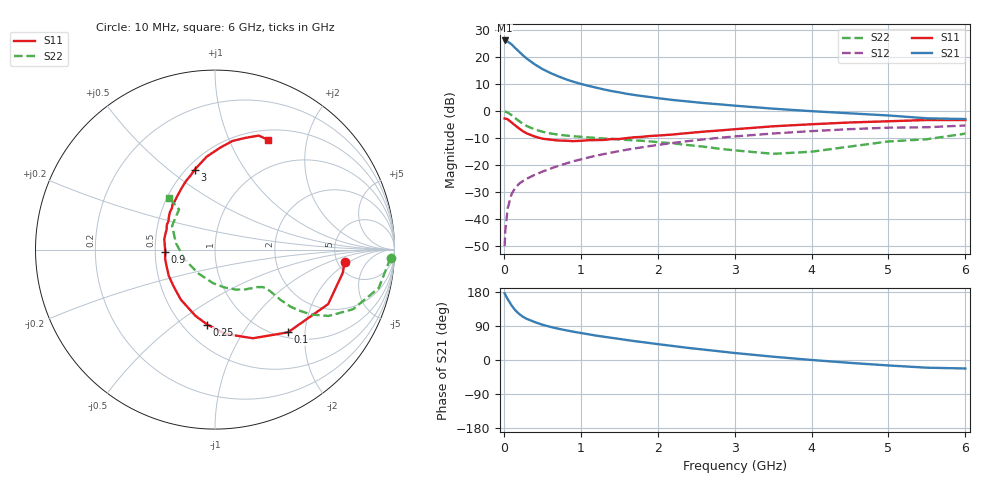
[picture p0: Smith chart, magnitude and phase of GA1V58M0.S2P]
! Infineon Technologies  Discrete & RF Semiconductors
! BF775
! Si NPN RF Bipolar Junction Transistor in SOT23
! VCE = 1.5 V  IC = 8 mA
! Common Emitter S-Parameters:  May  1996
# GHz  S  MA  R  50
!  f  S11  S21  S12  S22
! GHz  MAG  ANG  MAG  ANG  MAG  ANG  MAG  ANG
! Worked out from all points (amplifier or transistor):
!   36 points, 10 MHz to 6 GHz, reference 50 ohm
!   highest |S21| = 26.0 dB at 10 MHz (marker M1)
!   |S21| within 3 dB of that: start of sweep to 155.9 MHz
!   unconditionally stable (mu >= 1): 580.8 MHz to 4.246 GHz; 5.163 GHz to end of sweep
!   at 250 MHz: K = 0.65, MSG = 23.1 dB, |S12| = -25.8 dB
!   at 1.4 GHz: K = 1.14, MAG = 9.0 dB, |S12| = -15.4 dB
!   at 6 GHz: K = 1.00, MAG = 0.9 dB, |S12| = -5.4 dB
!   S11 on the Smith chart (normalised r, x): 10 MHz: 5.82, -1.65; 100 MHz: 1.10, -1.63; 250 MHz: 0.65, -0.66; 900 MHz: 0.57, -0.02; 3 GHz: 0.55, +0.62; 6 GHz: 0.62, +1.41
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0.01  0.7259 -5.3  19.96 176.0  0.0032 91.1  0.9804 -2.7
0.02  0.7233 -10.4  19.72 171.8  0.0064 85.4  0.9646 -5.4
0.05  0.6999 -25.7  19.03 160.6  0.016 77.7  0.9372 -13.2
0.1  0.6145 -48.6  16.93 144.1  0.0291 68.5  0.8373 -23.4
0.15  0.5371 -66.9  14.39 131.0  0.0385 62.3  0.733 -30.3
0.2  0.4732 -82.9  12.33 121.4  0.0455 59.4  0.6469 -34.0
0.25  0.4199 -95.9  10.58 113.9  0.0513 57.6  0.5756 -36.0
0.3  0.3849 -106.4  9.194 108.4  0.0564 57.6  0.5248 -37.1
0.4  0.3375 -124.4  7.262 100.2  0.0662 57.8  0.4578 -37.5
0.5  0.3079 -138.8  5.94 93.1  0.0757 58.5  0.4138 -37.2
0.6  0.2961 -150.5  5.051 87.7  0.0856 59.4  0.3855 -37.0
0.7  0.2851 -161.4  4.391 82.9  0.0958 60.3  0.3669 -37.1
0.9  0.2772 -177.3  3.47 74.8  0.1177 60.0  0.3418 -37.9
1.1  0.2884 168.4  2.904 67.9  0.1386 59.8  0.325 -40.1
1.3  0.2916 157.9  2.492 61.4  0.1602 58.6  0.3104 -42.5
1.6  0.3158 144.3  2.068 52.6  0.1926 56.2  0.2917 -47.9
2.2  0.3678 124.3  1.59 36.9  0.257 50.1  0.2524 -62.1
3  0.4599 104.2  1.252 18.5  0.3385 40.1  0.1873 -93.3
3.5  0.5206 95.0  1.101 8.7  0.3834 33.3  0.1619 -125.4
4.5  0.6128 80.9  0.903 -7.6  0.4615 19.8  0.2205 170.7
5.5  0.6803 69.0  0.731 -20.3  0.4996 5.6  0.3004 131.8
6  0.6791 64.1  0.709 -22.4  0.5388 1.6  0.3819 131.6
